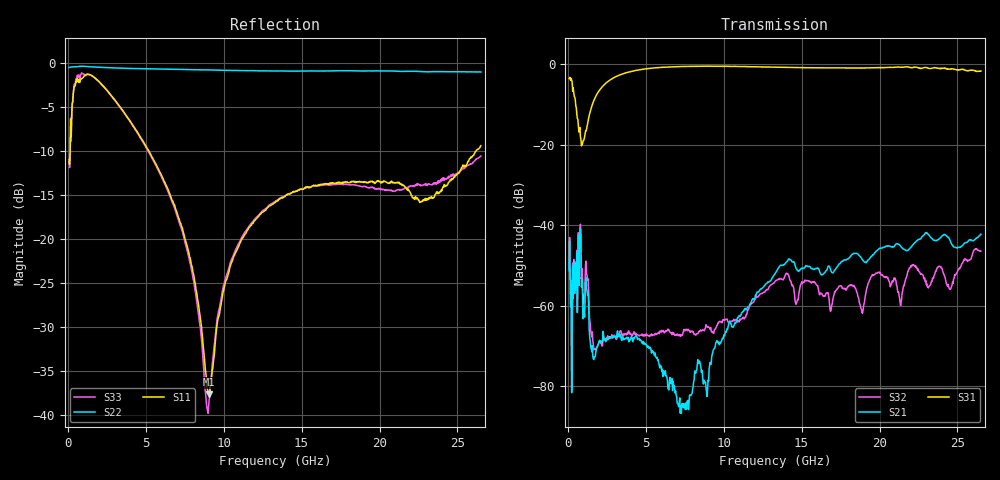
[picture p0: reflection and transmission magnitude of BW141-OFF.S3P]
!  3-Port S-parameters saved by WinCal
! VAR MeasName=S-Parameters (CALIBRATED_DATA) read from VNA (N5242A)
! VAR MeasDate=2014-8-25 14:20:30
! VAR NAME=1 2
! VAR FILENAME=1 2.S3P
! VAR DATE=2014-8-25 14:20:30
! VAR PHYS_PORTS=1,2,3
# Hz S MA R 50
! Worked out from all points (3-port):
!   801 points, 100 MHz to 26.5 GHz, reference 50 ohm
!   strongest paths, dB at 100 MHz, 6.7 GHz, 13.3 GHz, 19.9 GHz, 26.5 GHz:
!     S31: -3.6, -0.6, -0.7, -0.8, -1.7
!     S21: -51.4, -78.1, -52.1, -46.1, -42.2
!     S32: -50.5, -67.2, -54.0, -51.8, -46.4
!   lowest |S11| = -37.6 dB at 9.043 GHz (marker M1), VSWR 1.03, Z = 51.2 - j0.609 ohm
!   |S11| at or under -10 dB: start of sweep to 166.1 MHz; 5.226 GHz to 26.16 GHz (20.94 GHz wide, 133 % of centre)
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1e8  0.2844 -170.3  0.002718 -72.6  0.6641 -3.7
     0.002698 -72.5  0.9481 -179.8  0.002961 -71.6
     0.6641 -3.7  0.002996 -71.8  0.2773 -172.7
9.58e8  0.8274 177.9  0.001483 104.3  0.1033 3.5
        0.001498 103.9  0.9654 177.6  0.002148 124.0
        0.1034 3.5  0.002134 123.5  0.8752 174.5
1.783e9  0.8249 150.1  0.0002434 85.6  0.3908 51.1
         0.000237 85.0  0.9541 175.2  0.0002797 47.3
         0.3911 51.1  0.0002827 47.6  0.8212 147.5
4.456e9  0.41 100.8  0.0003981 28.4  0.8457 6.2
         0.0003969 29.0  0.9352 169.4  0.0004539 -18.1
         0.8456 6.0  0.0004358 -19.6  0.4053 97.1
6.865e9  0.1559 72.2  9.349e-05 -3.4  0.9354 -20.8
         9.328e-05 -6.1  0.9267 164.4  0.0004423 -68.0
         0.9341 -20.9  0.0004304 -69.7  0.1504 70.4
9.043e9  0.01317 -26.9  0.0001279 -143.3  0.9476 -40.2
         0.0001153 -143.5  0.9185 160.1  0.0005501 -109.6
         0.9492 -40.3  0.0005442 -112.0  0.01127 150.1
1.0429e10  0.07025 -118.9  0.0006315 -168.7  0.9414 -51.4
           0.0006392 -166.5  0.913 157.3  0.0006451 -129.3
           0.9422 -51.4  0.0006253 -127.0  0.07364 -155.9
1.33e10  0.1616 -141.3  0.002463 -172.9  0.9203 -72.2
         0.002496 -172.1  0.9068 151.6  0.002009 -167.3
         0.9235 -72.2  0.002004 -168.5  0.1637 -175.8
1.8877e10  0.2109 -161.7  0.003788 126.2  0.9 -109.0
           0.003781 127.6  0.9063 139.9  0.0008066 136.4
           0.9009 -109.0  0.0008191 131.7  0.1992 130.6
2.65e10  0.3406 -133.8  0.00759 105.5  0.7965 -171.1
         0.00776 108.9  0.8942 121.8  0.004683 110.0
         0.8244 -171.1  0.004765 105.3  0.2976 -28.0
